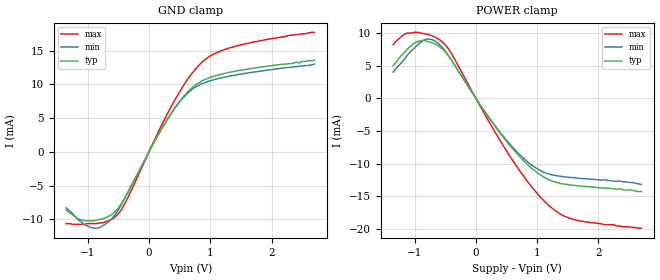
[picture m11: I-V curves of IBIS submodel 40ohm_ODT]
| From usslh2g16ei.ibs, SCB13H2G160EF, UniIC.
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| SUBMODEL 40ohm_ODT
[Submodel]   40ohm_ODT
Submodel_type  Dynamic_clamp
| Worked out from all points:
|   GND clamp passes 1 mA (typ) near -0.06 V on its own axis
|   POWER clamp passes 1 mA (typ) near -0.07 V on its own axis
[GND Clamp]
|Voltage   I(typ)   I(min)   I(max)
-1.35V    -8.6mA     -8.3mA     -10.63mA
-1.2V     -9.7mA     -9.6mA     -10.73mA
-950mV    -10.2mA    -11.2mA    -10.63mA
-800mV    -10mA      -11.2mA    -10.52mA
-650mV    -9.52mA    -10.29mA   -10.2mA
-400mV    -6.89mA    -6.98mA    -7.771mA
100mV     1.707mA    1.705mA    1.963mA
400mV     6.238mA    6.182mA    7.329mA
650mV     9.06mA     8.86mA     11mA
950mV     10.86mA    10.39mA    13.91mA
1.45V     12.03mA    11.45mA    15.75mA
2.7V      13.6mA     13mA       17.71mA
[POWER Clamp]
|Voltage   I(typ)   I(min)   I(max)
-1.35V    5mA        4mA        8.229mA
-1.15V    7.2mA      6.2mA      9.896mA
-1V       8.5mA      7.7mA      10.1mA
-850mV    8.9mA      8.9mA      9.896mA
-700mV    8.46mA     8.93mA     9.521mA
-400mV    5.886mA    5.893mA    6.896mA
150mV     -2.112mA   -2.075mA   -2.532mA
550mV     -7.172mA   -6.963mA   -8.792mA
900mV     -10.64mA   -10.14mA   -13.43mA
1.2V      -12.5mA    -11.62mA   -16.49mA
1.65V     -13.39mA   -12.22mA   -18.69mA
2.7V      -14.3mA    -13.2mA    -19.9mA
